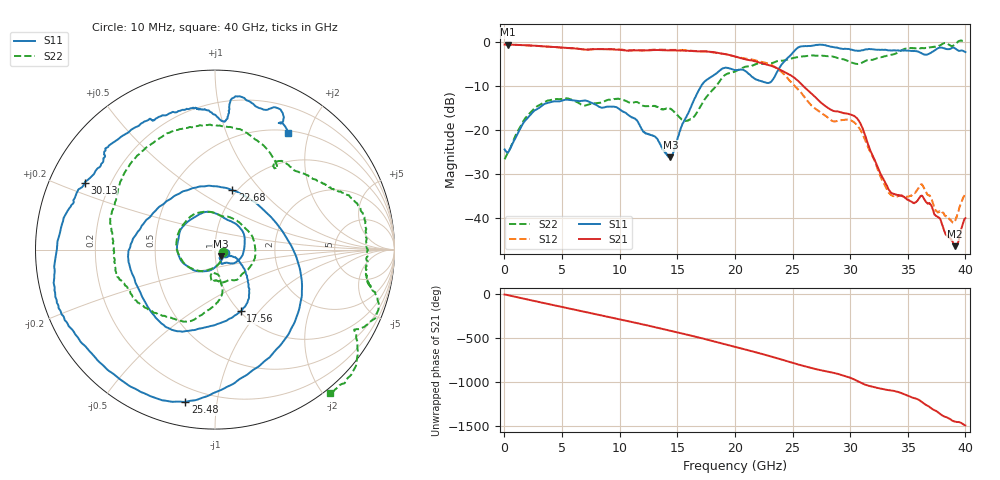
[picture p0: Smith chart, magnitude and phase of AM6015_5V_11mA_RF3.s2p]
!Agilent Technologies,E8364B,MY43040894,A.07.50.67
!Agilent E8364B: A.07.50.67
!Date: Wednesday, May 01, 2019 08:20:51
!Correction: S11(Full 2 Port(1,2))
!S21(Full 2 Port(1,2))
!S12(Full 2 Port(1,2))
!S22(Full 2 Port(1,2))
!S2P File: Measurements: S11, S21, S12, S22:
# Hz S  dB  R 50
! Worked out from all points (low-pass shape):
!   1601 points, 10 MHz to 40 GHz, reference 50 ohm
!   highest |S21| = -0.61 dB at 284.9 MHz (marker M1); lowest = -46.3 dB at 39.1 GHz (marker M2)
!   |S21| within 3 dB of the highest: start of sweep to 20.38 GHz
!   lowest |S11| = -26.1 dB at 14.41 GHz (marker M3), VSWR 1.10, Z = 53.2 - j4 ohm
!   |S11| at or under -10 dB: start of sweep to 17.08 GHz
!   |S22| runs from -26.6 to 0.3 dB; largest |S21 - S12| = 0.094
!   S11 on the Smith chart (normalised r, x): 10 MHz: 1.12, -0.04; 17.56 GHz: 1.01, -0.81; 22.68 GHz: 0.95, +0.71; 25.48 GHz: 0.12, -0.82; 30.13 GHz: 0.11, +0.24; 40 GHz: 0.53, +1.68
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1e7  -24.37 -18.4  -0.62 -2.0  -0.52 -1.8  -26.59 -13.7
2.849312e8  -25.13 -27.2  -0.61 -8.5  -0.60 -8.5  -25.06 -30.0
3.2092e9  -14.55 -154.0  -0.98 -93.0  -0.99 -93.1  -14.06 -167.2
5.058738e9  -13.26 157.0  -1.29 -145.4  -1.35 -145.2  -12.88 133.9
6.683331e9  -13.37 115.9  -1.66 168.8  -1.66 169.2  -14.25 83.1
9.732569e9  -14.85 26.3  -1.77 82.7  -1.69 83.1  -12.90 -7.0
1.168208e10  -18.62 -41.6  -1.95 27.2  -1.88 27.3  -13.87 -57.5
1.335666e10  -22.47 -64.3  -1.85 -22.1  -1.77 -22.2  -14.92 -82.4
1.44064e10  -26.13 -49.4  -1.94 -54.0  -1.83 -54.3  -15.12 -96.4
1.588103e10  -16.47 -25.6  -2.01 -100.2  -1.95 -101.1  -17.79 -94.9
1.755561e10  -8.57 -67.3  -2.20 -154.2  -2.15 -155.5  -12.42 -80.1
2.0005e10  -6.40 -152.4  -3.32 121.6  -3.33 121.3  -6.70 -126.0
2.117971e10  -7.24 165.3  -4.10 82.4  -3.91 81.6  -5.56 -151.1
2.267933e10  -9.26 73.7  -5.10 29.2  -4.76 25.6  -5.01 -178.5
2.407898e10  -5.07 -31.1  -6.54 -23.5  -6.88 -33.3  -4.27 157.8
2.547863e10  -1.27 -101.0  -8.83 -77.9  -10.76 -83.8  -3.44 133.7
2.667833e10  -0.88 -144.2  -11.76 -119.8  -14.48 -118.5  -3.08 110.2
3.012747e10  -1.77 152.8  -16.55 123.9  -17.87 138.5  -4.69 53.7
3.335166e10  -1.95 115.8  -33.45 -10.6  -34.19 13.8  -3.03 31.8
3.622594e10  -2.65 88.9  -34.84 -146.5  -32.30 -127.5  -1.38 -4.4
3.910022e10  -1.47 63.3  -46.27 -8.9  -40.49 20.8  -0.61 -32.3
4e10  -2.31 57.8  -39.91 -52.4  -34.59 -47.9  0.21 -51.4
